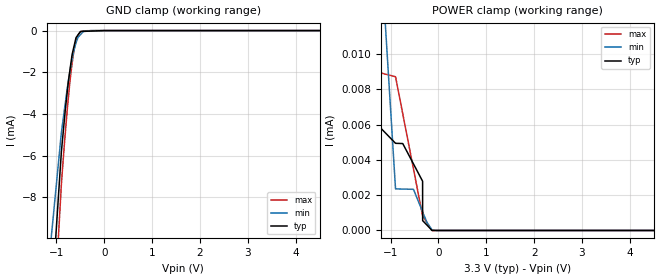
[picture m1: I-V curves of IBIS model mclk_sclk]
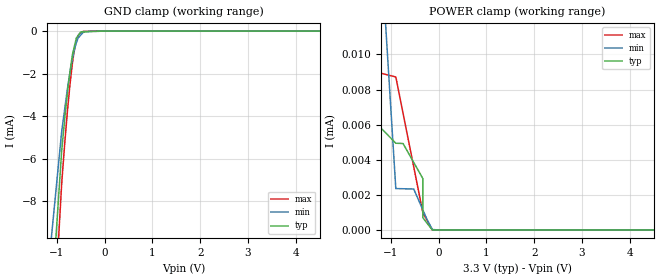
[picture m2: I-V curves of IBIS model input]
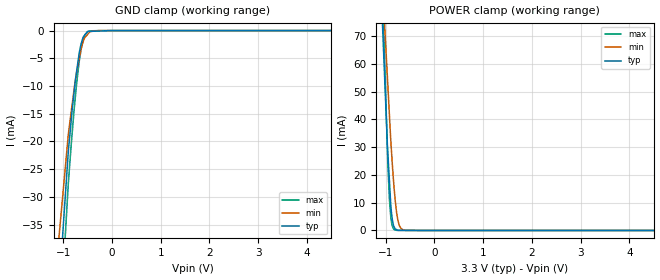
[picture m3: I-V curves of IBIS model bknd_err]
|Texas Instruments Incorporated
| 8-Channel HD Compatible Audio Processor with PWM Output
| Marketing part#   Digital Voltage Range   Package-type   #pins
| TAS5548DGG   3.0V - 3.6V   PSOP   56
| TAS5548DGGR   3.0V - 3.6V   PSOP   56
[IBIS Ver]   4.0
[File name]   tas5548.ibs
[File Rev]   1.0
[Date]   8/2/2012
[Source]
| Texas Instruments Incorporated.
| Analog-eLab Design Center, HPA
| 12500 TI Blvd
| Dallas, TX -75243
| e-mail: elab_scm_ibis@list.ti.com
[Notes]   Revision History:
| Rev 1.1: 8/2/2012
| - addtioanl models, xtalo, xtali and lrcklo added per request.
| - Non-monotonic behavior warning for lrclko is minor and can
|   be ignored safely.
| Rev 1.0: 7/30/2012
| - Initial version of the model
| - Model generated from simulations in TISPICE
| - Model matched to SPICE simulation
| - C_comp although listed in numerical order of value are
|   obtained from varying PVT conditions. For PVT conditions for
|   each specific value refer the buffer description under
|   respective [Model]. IBIS model user is responsible for using
|   appropriate C_comp to simulate for Signal Integrity.
[Disclaimer]
| This model is designed as an aid for customers of Texas Instruments.
| TI and its licensors and suppliers make no warranties, either expressed
| or implied, with respect to this  model, including the warranties of
| merchantability or fitness for a particular purpose. The model is
| provided solely on an "as is" basis. The entire risk as to its quality
| and performance is with the customer.
[Copyright]
 (C) Copyright 2012 Texas Instruments Incorporated.All rights reserved.
|   TAS5548
[Component]   TAS5548
[Manufacturer]   TI
[Package]   |56 PSOP   -  DCA package
|   typ   min   max
R_pkg   0.1   0.1   0.1
L_pkg   1.0nH   1.0nH   1.0nH
C_pkg   0.4pF   0.4pF   0.4pF
[Pin]  signal_name   model_name   R_pin   L_pin   C_pin
1   PWM_HPM_L   output   NA   NA   NA
2   PWM_HPP_L   output   NA   NA   NA
3   PWM_HPM_R   output   NA   NA   NA
4   PWM_HPP_R   output   NA   NA   NA
5   AVSS   gnd   NA   NA   NA
6   PLL_FLTM   term   NA   NA   NA
7   PLL_FLTP   term   NA   NA   NA
8   VR_ANA   power   NA   NA   NA
9   AVDD   power   NA   NA   NA
10   ASEL_EMO2   asel_emo2   NA   NA   NA
11   XTALI   xtali   NA   NA   NA
12   XTALO   xtalo   NA   NA   NA
13   DVSS2_CORE   gnd   NA   NA   NA
14   DVDD2_CORE   power   NA   NA   NA
15   EMO1   output   NA   NA   NA
16   _RESET   input   NA   NA   NA
17   _HP_SEL   input   NA   NA   NA
18   _PDN   input   NA   NA   NA
19   _MUTE   input   NA   NA   NA
20   SDA   sda   NA   NA   NA
21   SCL   input   NA   NA   NA
22   LRCLK   input   NA   NA   NA
23   SCLK   mclk_sclk   NA   NA   NA
24   SDIN1   sdin1   NA   NA   NA
25   SDIN2   input   NA   NA   NA
26   SDIN2_1   input   NA   NA   NA
27   SDIN2_2   input   NA   NA   NA
28   VR_DIG   power   NA   NA   NA
29   SDOUT   lrclko   NA   NA   NA
30   SCLKO   lrclko   NA   NA   NA
31   LRCLKO   lrclko   NA   NA   NA
32   TEST   test   NA   NA   NA
33   PSVC/MLCK   output   NA   NA   NA
34   _BKND_ERR   bknd_err   NA   NA   NA
35   DVDD1_CORE   power   NA   NA   NA
36   DVSS2_CORE   gnd   NA   NA   NA
37   VALID   valid   NA   NA   NA
38   PWM_M_1   output   NA   NA   NA
39   PWM_P_1   output   NA   NA   NA
40   PWM_M_2   output   NA   NA   NA
41   PWM_P_2   output   NA   NA   NA
42   PWM_M_3   output   NA   NA   NA
43   PWM_P_3   output   NA   NA   NA
44   PWM_M_4   output   NA   NA   NA
45   PWM_P_4   output   NA   NA   NA
46   PWM_M_7   output   NA   NA   NA
47   PWM_P_7   output   NA   NA   NA
48   PWM_M_8   output   NA   NA   NA
49   PWM_P_8   output   NA   NA   NA
50   AVDD_PWM   gnd   NA   NA   NA
51   AVSS_PWM   power   NA   NA   NA
52   VR_PWM   term   NA   NA   NA
53   PWM_M_5   output   NA   NA   NA
54   PWM_P_5   output   NA   NA   NA
55   PWM_M_6   output   NA   NA   NA
56   PWM_P_6   output   NA   NA   NA
[Model] term
Model_type Terminator
C_comp   1.0e-20F  1.0e-20F  1.0e-20F
|   typ   min   max
[Voltage Range]   3.3V   3.0V   3.6V
[POWER Clamp Reference]   3.3V   3.0V   3.6V
[GND Clamp Reference]   0V   0V   0V
|Ambient Temperature   27   125   0
|Junction Temperature
[Temperature Range]   27   125   0
| Models and submodels in the file (13): mclk_sclk (Input), input (Input), bknd_err (Input), test (Input), sdin1 (Input), valid (3-state), output (3-state), asel_emo2 (I/O), sda (I/O), xtalo (Output), xtali (Input), lrclko (I/O), term (Terminator)
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|   mclk_sclk Model
[Model]   mclk_sclk
Model_type   Input
Vinl = 0.8
Vinh = 2.0
|   typ   min   max
|   (nom PVT)   (fast PVT)   (slow PVT)
|C_comp from frequency sweep method (F=50MHz)
|Average
|C_comp   2.253e-12   2.203e-12   2.284e-12
|C_comp from LC tank measurement(L=1nH)
|Average
|Resonant Frequency(Hz)   5.390e+09   5.790e+09   5.310e+09
C_comp   8.728e-13   7.563e-13   8.993e-13
| Where nom  PVT is Nominal Process, 3.3V, 27C
|   Fast PVT is Strong Process,  3.6V, 0C
|   Slow PVT is Weak Process,   3V, 125C
[Voltage Range]   3.3   3   3.6
|Ambient Temperature   27   125   0
|Junction Temperature
[Temperature Range]   27   125   0
[Power Clamp Reference]   3.3   3   3.6
[GND Clamp Reference]   0   0   0
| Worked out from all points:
|   GND clamp passes 1 mA (typ) near -0.66 V on its own axis
|   POWER clamp passes 1 mA (typ) near -3.28 V on its own axis
[GND Clamp]
|   Voltage   I(typ)   I(min)   I(max)
-3.3V     -1.87A     -1.609A    -1.97A
-1.58V    -29.61mA   -21.11mA   -35.32mA
-897.6mV  -5.812mA   -4.894mA   -7.371mA
-777.6mV  -2.997mA   -2.824mA   -3.87mA
-727.2mV  -2.035mA   -2.082mA   -2.648mA
-676.8mV  -1.206mA   -1.427mA   -1.628mA
-630mV    -722.2uA   -907.1uA   -900.7uA
-590.4mV  -334.7uA   -574.9uA   -473.3uA
-498.3mV  -43.55uA   -194.5uA   -65.94uA
-438mV    -38.25uA   -41.94uA   -11.17uA
-285mV    -24.79uA   -1.199uA   -5.561uA
6.6V      0A         0A         0A
[POWER Clamp]
|   Voltage   I(typ)   I(min)   I(max)
-3.3V     1.043mA    5.986mA    1.052mA
-2.262V   46.15uA    205.9uA    27.66uA
-2.164V   27.73uA    164.8uA    11.19uA
-2.059V   8.187uA    121.1uA    9.525uA
-1.878V   7.681uA    45.34uA    9.4uA
-896.4mV  4.943uA    2.358uA    8.717uA
-745.8mV  4.927uA    2.348uA    6.615uA
-522mV    3.775uA    2.334uA    3.491uA
-331.2mV  2.793uA    1.061uA    828.1nA
-330mV    557.6nA    1.053uA    823.1nA
-133.2mV  0A         23.77nA    0A
6.6V      0A         0A         0A
|   input Model
[Model]   input
Model_type   Input
Vinl = 0.8
Vinh = 2
|   typ   min   max
|   (nom PVT)   (fast PVT)   (slow PVT)
|C_comp from frequency sweep method (F=50MHz)
|Average
|C_comp   1.652e-12   1.610e-12   1.681e-12
|C_comp from LC tank measurement(L=1nH)
|Average
|Resonant Frequency(Hz)   5.790e+09   6.190e+09   5.760e+09
C_comp   7.563e-13   6.617e-13   7.642e-13
| Where nom  PVT is Nominal Process, 3.3V, 27C
|   Fast PVT is Strong Process,  3.6V, 0C
|   Slow PVT is Weak Process,   3V, 125C
[Voltage Range]   3.3   3   3.6
|Ambient Temperature   27   125   0
|Junction Temperature
[Temperature Range]   27   125   0
[Power Clamp Reference]   3.3   3   3.6
[GND Clamp Reference]   0   0   0
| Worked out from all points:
|   GND clamp passes 1 mA (typ) near -0.66 V on its own axis
|   POWER clamp passes 1 mA (typ) near -3.28 V on its own axis
[GND Clamp]
|   Voltage   I(typ)   I(min)   I(max)
-3.3V     -1.857A    -1.601A    -1.955A
-1.58V    -28.79mA   -20.52mA   -34.35mA
-897.6mV  -5.65mA    -4.735mA   -7.189mA
-777.6mV  -2.933mA   -2.726mA   -3.785mA
-745.8mV  -2.281mA   -2.263mA   -3.034mA
-676.8mV  -1.177mA   -1.373mA   -1.595mA
-630mV    -704.8uA   -870.1uA   -881.6uA
-590.4mV  -326.4uA   -550uA     -463uA
-498.3mV  -42.38uA   -187.1uA   -64.44uA
-441mV    -37.47uA   -42.7uA    -12.29uA
-285mV    -24.12uA   -1.155uA   -5.432uA
6.6V      0A         0A         0A
[POWER Clamp]
|   Voltage   I(typ)   I(min)   I(max)
-3.3V     1.043mA    5.986mA    1.052mA
-2.262V   46.15uA    205.9uA    27.66uA
-2.164V   27.73uA    164.8uA    11.19uA
-2.059V   8.187uA    121.1uA    9.525uA
-1.878V   7.681uA    45.34uA    9.399uA
-896.4mV  4.943uA    2.359uA    8.717uA
-745.8mV  4.927uA    2.349uA    6.656uA
-522mV    3.849uA    2.335uA    3.592uA
-331.2mV  2.93uA     1.146uA    980nA
-330mV    689.6nA    1.138uA    974.1nA
-133.2mV  0A         31.93nA    0A
6.6V      0A         0A         0A
|   bknd_err Model
[Model]   bknd_err
Model_type   Input
Vinl = 0.8
Vinh = 2.0
|   typ   min   max
|   (nom PVT)   (fast PVT)   (slow PVT)
|C_comp from frequency sweep method (F=50MHz)
|Average
|C_comp   1.392e-12   1.371e-12   1.400e-12
|C_comp from LC tank measurement(L=1nH)
|Average
|Resonant Frequency(Hz)   4.830e+09   4.870e+09   4.820e+09
C_comp   1.087e-12   1.069e-12   1.091e-12
| Where nom  PVT is Nominal Process, 3.3V, 27C
|   Fast PVT is Strong Process,  3.6V, 0C
|   Slow PVT is Weak Process,   3V, 125C
[Voltage Range]   3.3   3   3.6
|Ambient Temperature   27   125   0
|Junction Temperature
[Temperature Range]   27   125   0
[Power Clamp Reference]   3.3   3   3.6
[GND Clamp Reference]   0   0   0
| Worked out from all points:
|   GND clamp passes 1 mA (typ) near -0.58 V on its own axis
|   POWER clamp passes 1 mA (typ) near -0.82 V on its own axis
[GND Clamp]
|   Voltage   I(typ)   I(min)   I(max)
-3.3V     -1.791A    -1.554A    -1.888A
-1.541V   -105.7mA   -80.99mA   -125.6mA
-897.6mV  -21.93mA   -18.81mA   -27.74mA
-818.4mV  -14.4mA    -13.37mA   -18.61mA
-781.2mV  -11.41mA   -10.82mA   -14.67mA
-745.8mV  -8.557mA   -8.651mA   -11.39mA
-680.4mV  -4.536mA   -5.262mA   -6.091mA
-633.6mV  -2.386mA   -3.339mA   -3.343mA
-594mV    -1.228mA   -2.043mA   -1.749mA
-501.6mV  -159.2uA   -704.3uA   -241.6uA
-285mV    -90uA      -3.941uA   -18.71uA
6.6V      0A         0A         0A
[POWER Clamp]
|   Voltage   I(typ)   I(min)   I(max)
-3.3V     1.273A     949.3mA    1.894A
-1.063V   72.06mA    86.95mA    87.55mA
-1.04V    62.51mA    79.63mA    71.76mA
-957.6mV  27.98mA    52.35mA    23.88mA
-925.2mV  17.91mA    41.67mA    11.33mA
-884.4mV  6.709mA    29mA       3.287mA
-858mV    3.117mA    21.97mA    1.24mA
-817.2mV  920.9uA    12.97mA    228.2uA
-771mV    253.2uA    5.628mA    35.57uA
-723mV    45.66uA    1.855mA    5.78uA
-591mV    37.29uA    54.53uA    2.421uA
6.6V      0A         0A         0A
